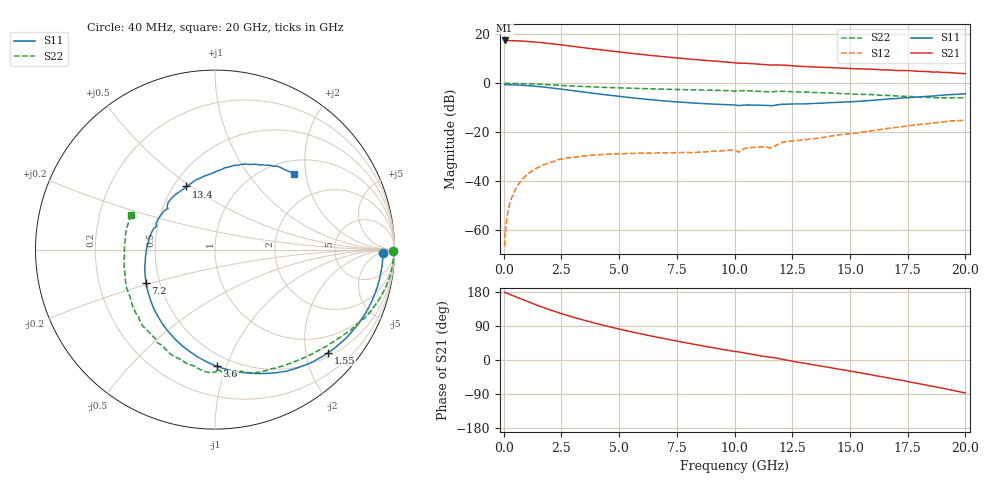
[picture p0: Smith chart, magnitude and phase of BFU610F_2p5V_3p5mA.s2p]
! Filename:  P:\Prog\Test\Noise\ATS_data\Testdata_Net\SplitFiles\BFU610_2W_A5_HighFreq_2.5V_3.5mA_D.s2p
! Date/Time: Wed 10/Aug/2011 16:55:19
! BFU610_2W_A5_HighFreq_Bias3_2.5V_1mA_10mA_R.s2p
! MDIF S-parameter v. bias file
! BFU610_2W_A5_HighFreq_2.5V_1mA_10mA
! Date/time Mon Aug 08 14:04:20 2011
! VAR V_out= 2.5000
! VAR I_out= 3.5050
! VAR V_in= 0.8845
! VAR I_in= 0.0272
! Device data file deembeded for feedlines and parallel
! Original file: \SplitFiles\BFU610_2W_A5_HighFreq_2.5V_3.5mA_R.s2p
! Feed-files: PR003V01_101208_Feed1.s2p, PR003V01_101208_Feed2.s2p
! Parallel-file: PR003V01_101208_Par.s2p
# MHz S MA R 50
!  Freq-MHz  S11-mag  S11-arg  S21-mag  S21-arg  S12-mag  S12-arg  S22-mag  S22-arg
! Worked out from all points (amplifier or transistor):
!   167 points, 40 MHz to 20 GHz, reference 50 ohm
!   highest |S21| = 17.5 dB at 40 MHz (marker M1)
!   |S21| within 3 dB of that: start of sweep to 3.494 GHz
!   unconditionally stable (mu >= 1): 5.737 GHz to 17.46 GHz
!   at 550 MHz: K = 0.03, MSG = 29.9 dB, |S12| = -42.5 dB
!   at 4.2 GHz: K = 0.69, MSG = 21.4 dB, |S12| = -29.1 dB
!   at 20 GHz: K = 0.82, MSG = 9.5 dB, |S12| = -15.1 dB
!   S11 on the Smith chart (normalised r, x): 40 MHz: 28, -8; 1.55 GHz: 0.59, -2.46; 3.6 GHz: 0.41, -0.93; 7.2 GHz: 0.42, -0.19; 13.4 GHz: 0.58, +0.48; 20 GHz: 1.27, +1.71
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40  0.9365 -1.1  7.466 178.6  0.0004736 85.6  0.9944 -0.3
50  0.9363 -1.3  7.432 178.7  0.0008978 116.2  0.9945 -0.5
180  0.9355 -5.0  7.405 175.4  0.002343 89.8  0.9956 -2.0
440  0.9287 -12.4  7.374 168.8  0.005956 85.6  0.9924 -5.2
950  0.9013 -26.5  7.185 156.2  0.01282 75.4  0.9781 -11.1
1550  0.8526 -42.3  6.794 142.3  0.01983 64.9  0.9528 -17.5
1950  0.8138 -52.5  6.507 133.5  0.0237 58.8  0.9338 -21.5
2350  0.7725 -62.1  6.177 125.3  0.02746 54.0  0.9097 -25.4
2900  0.7153 -74.3  5.738 114.8  0.0304 45.6  0.8831 -29.8
3400  0.6685 -84.9  5.355 106.2  0.03252 41.6  0.8596 -33.7
3600  0.6503 -89.1  5.217 102.9  0.0333 40.0  0.8505 -35.2
4400  0.5825 -104.6  4.689 90.3  0.0354 34.3  0.8224 -40.8
5000  0.5393 -115.8  4.348 81.7  0.03638 31.3  0.803 -44.8
5800  0.4907 -130.2  3.946 70.8  0.03721 28.7  0.782 -50.1
6800  0.4421 -147.4  3.525 58.3  0.03779 27.1  0.7595 -56.6
7200  0.4267 -154.2  3.384 53.5  0.03809 27.1  0.7514 -59.3
8600  0.3853 -177.1  2.969 37.5  0.03958 29.8  0.7291 -68.5
10200  0.35 158.1  2.565 21.2  0.0392 34.7  0.6944 -77.8
12000  0.3705 134.7  2.357 2.6  0.06089 43.3  0.6864 -92.0
13400  0.3868 114.5  2.151 -12.4  0.07363 34.5  0.6474 -105.4
16800  0.4816 77.0  1.862 -48.9  0.1224 17.7  0.5593 -144.6
20000  0.6087 44.0  1.569 -87.0  0.1763 -13.0  0.5048 157.8
